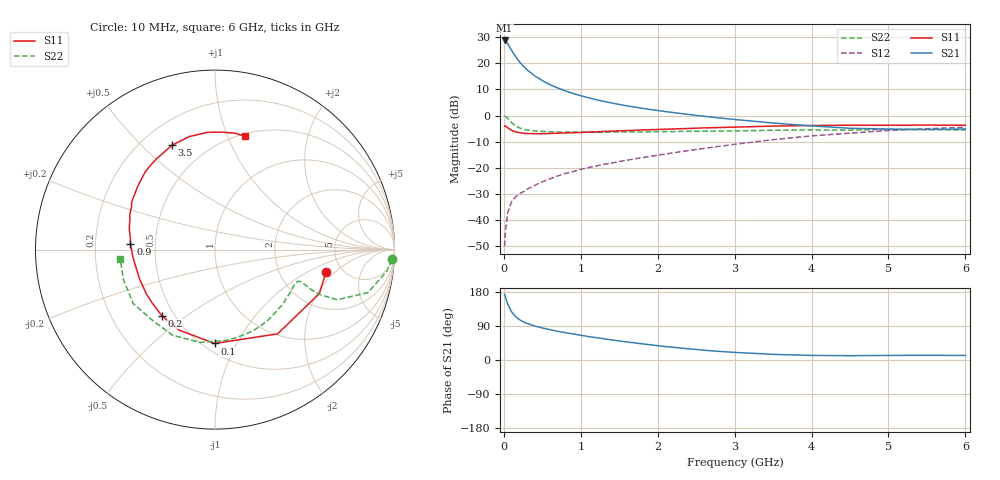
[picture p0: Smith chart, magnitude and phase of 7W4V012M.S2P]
! Infineon Technologies  Discrete & RF Semiconductors
! BFS17W
! Si NPN RF Bipolar Junction Transistor in SOT323
! VCE = 4 V  IC = 12 mA
! Common Emitter S-Parameters:  August  1999
# GHz  S  MA  R  50
!  f  S11  S21  S12  S22
! GHz  MAG  ANG  MAG  ANG  MAG  ANG  MAG  ANG
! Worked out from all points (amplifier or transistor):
!   36 points, 10 MHz to 6 GHz, reference 50 ohm
!   highest |S21| = 28.7 dB at 10 MHz (marker M1)
!   |S21| within 3 dB of that: start of sweep to 85.76 MHz
!   unconditionally stable (mu >= 1): 366.9 MHz to 2.363 GHz; 5.003 GHz to end of sweep
!   at 250 MHz: K = 0.85, MSG = 24.1 dB, |S12| = -29.1 dB
!   at 1.4 GHz: K = 1.19, MAG = 8.8 dB, |S12| = -18.1 dB
!   at 6 GHz: K = 1.06, MAG = -1.8 dB, |S12| = -4.4 dB
!   S11 on the Smith chart (normalised r, x): 10 MHz: 3.74, -1.55; 100 MHz: 0.57, -0.82; 200 MHz: 0.43, -0.40; 900 MHz: 0.36, +0.03; 3.5 GHz: 0.32, +0.62; 6 GHz: 0.52, +1.16
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0.01  0.6311 -11.4  27.23 173.3  0.0032 80.7  0.9858 -3.2
0.02  0.6308 -22.9  26.77 166.0  0.006 83.0  0.9648 -7.2
0.05  0.5848 -53.4  23.67 147.8  0.014 70.1  0.8848 -15.7
0.1  0.5231 -90.3  17.77 127.4  0.0225 59.9  0.7367 -22.3
0.15  0.4912 -114.2  13.56 114.8  0.0277 55.0  0.6383 -23.2
0.2  0.4728 -128.9  10.8 106.9  0.0319 55.7  0.5853 -22.7
0.25  0.4593 -139.8  8.889 101.1  0.0349 55.4  0.5511 -21.7
0.3  0.4548 -147.4  7.532 96.7  0.039 58.3  0.5323 -21.1
0.4  0.4511 -158.7  5.762 89.8  0.0464 60.7  0.508 -20.5
0.5  0.4506 -166.0  4.655 84.5  0.0545 62.6  0.4976 -20.7
0.6  0.455 -171.5  3.893 80.0  0.0619 64.3  0.4915 -21.5
0.7  0.4611 -176.3  3.369 75.9  0.0703 65.5  0.4869 -22.8
0.9  0.4725 176.1  2.644 68.7  0.0854 66.9  0.482 -26.2
1.1  0.4834 169.2  2.188 61.9  0.1016 67.8  0.4819 -30.3
1.3  0.4973 163.3  1.869 55.9  0.1171 68.4  0.4811 -35.1
1.6  0.5177 155.5  1.534 47.6  0.1403 69.3  0.4835 -42.4
2.2  0.5546 141.3  1.142 33.5  0.1944 70.0  0.4955 -59.2
2.8  0.591 127.5  0.902 22.7  0.2582 67.9  0.5048 -77.2
3.5  0.6292 112.3  0.721 14.9  0.3467 62.6  0.5236 -98.9
4.5  0.6546 93.7  0.572 11.4  0.4613 50.1  0.5263 -132.1
5.5  0.6582 80.4  0.543 12.4  0.5605 37.3  0.5369 -161.6
6  0.6538 75.1  0.554 12.0  0.5993 31.1  0.531 -174.6
